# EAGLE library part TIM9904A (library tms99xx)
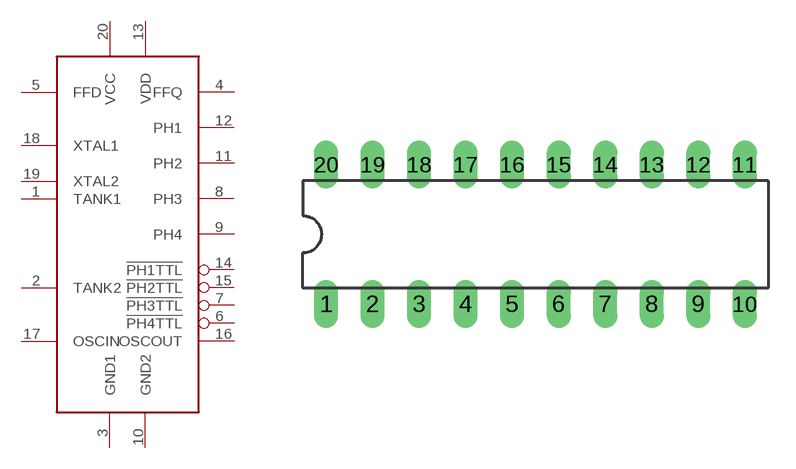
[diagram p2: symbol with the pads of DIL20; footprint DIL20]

Designator prefix -

## TIM9904A  [DIL20]
1  TANK1  in
2  TANK2  in
3  GND1  pwr
4  FFQ  out
5  FFD  in
6  !PH4TTL  out
7  !PH3TTL  out
8  PH3  out
9  PH4  out
10  GND2  pwr
11  PH2  out
12  PH1  out
13  VDD  pwr
14  !PH1TTL  out
15  !PH2TTL  out
16  OSCOUT  out
17  OSCIN  in
18  XTAL1  in
19  XTAL2  in
20  VCC  pwr

## Footprint DIL20 (pad centres in mm)
drill 0.813 long: 1 -11.43,-3.81; 2 -8.89,-3.81; 3 -6.35,-3.81; 4 -3.81,-3.81; 5 -1.27,-3.81; 6 1.27,-3.81; 7 3.81,-3.81; 8 6.35,-3.81; 9 8.89,-3.81; 10 11.43,-3.81; 11 11.43,3.81; 12 8.89,3.81; 13 6.35,3.81; 14 3.81,3.81; 15 1.27,3.81; 16 -1.27,3.81; 17 -3.81,3.81; 18 -6.35,3.81; 19 -8.89,3.81; 20 -11.43,3.81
